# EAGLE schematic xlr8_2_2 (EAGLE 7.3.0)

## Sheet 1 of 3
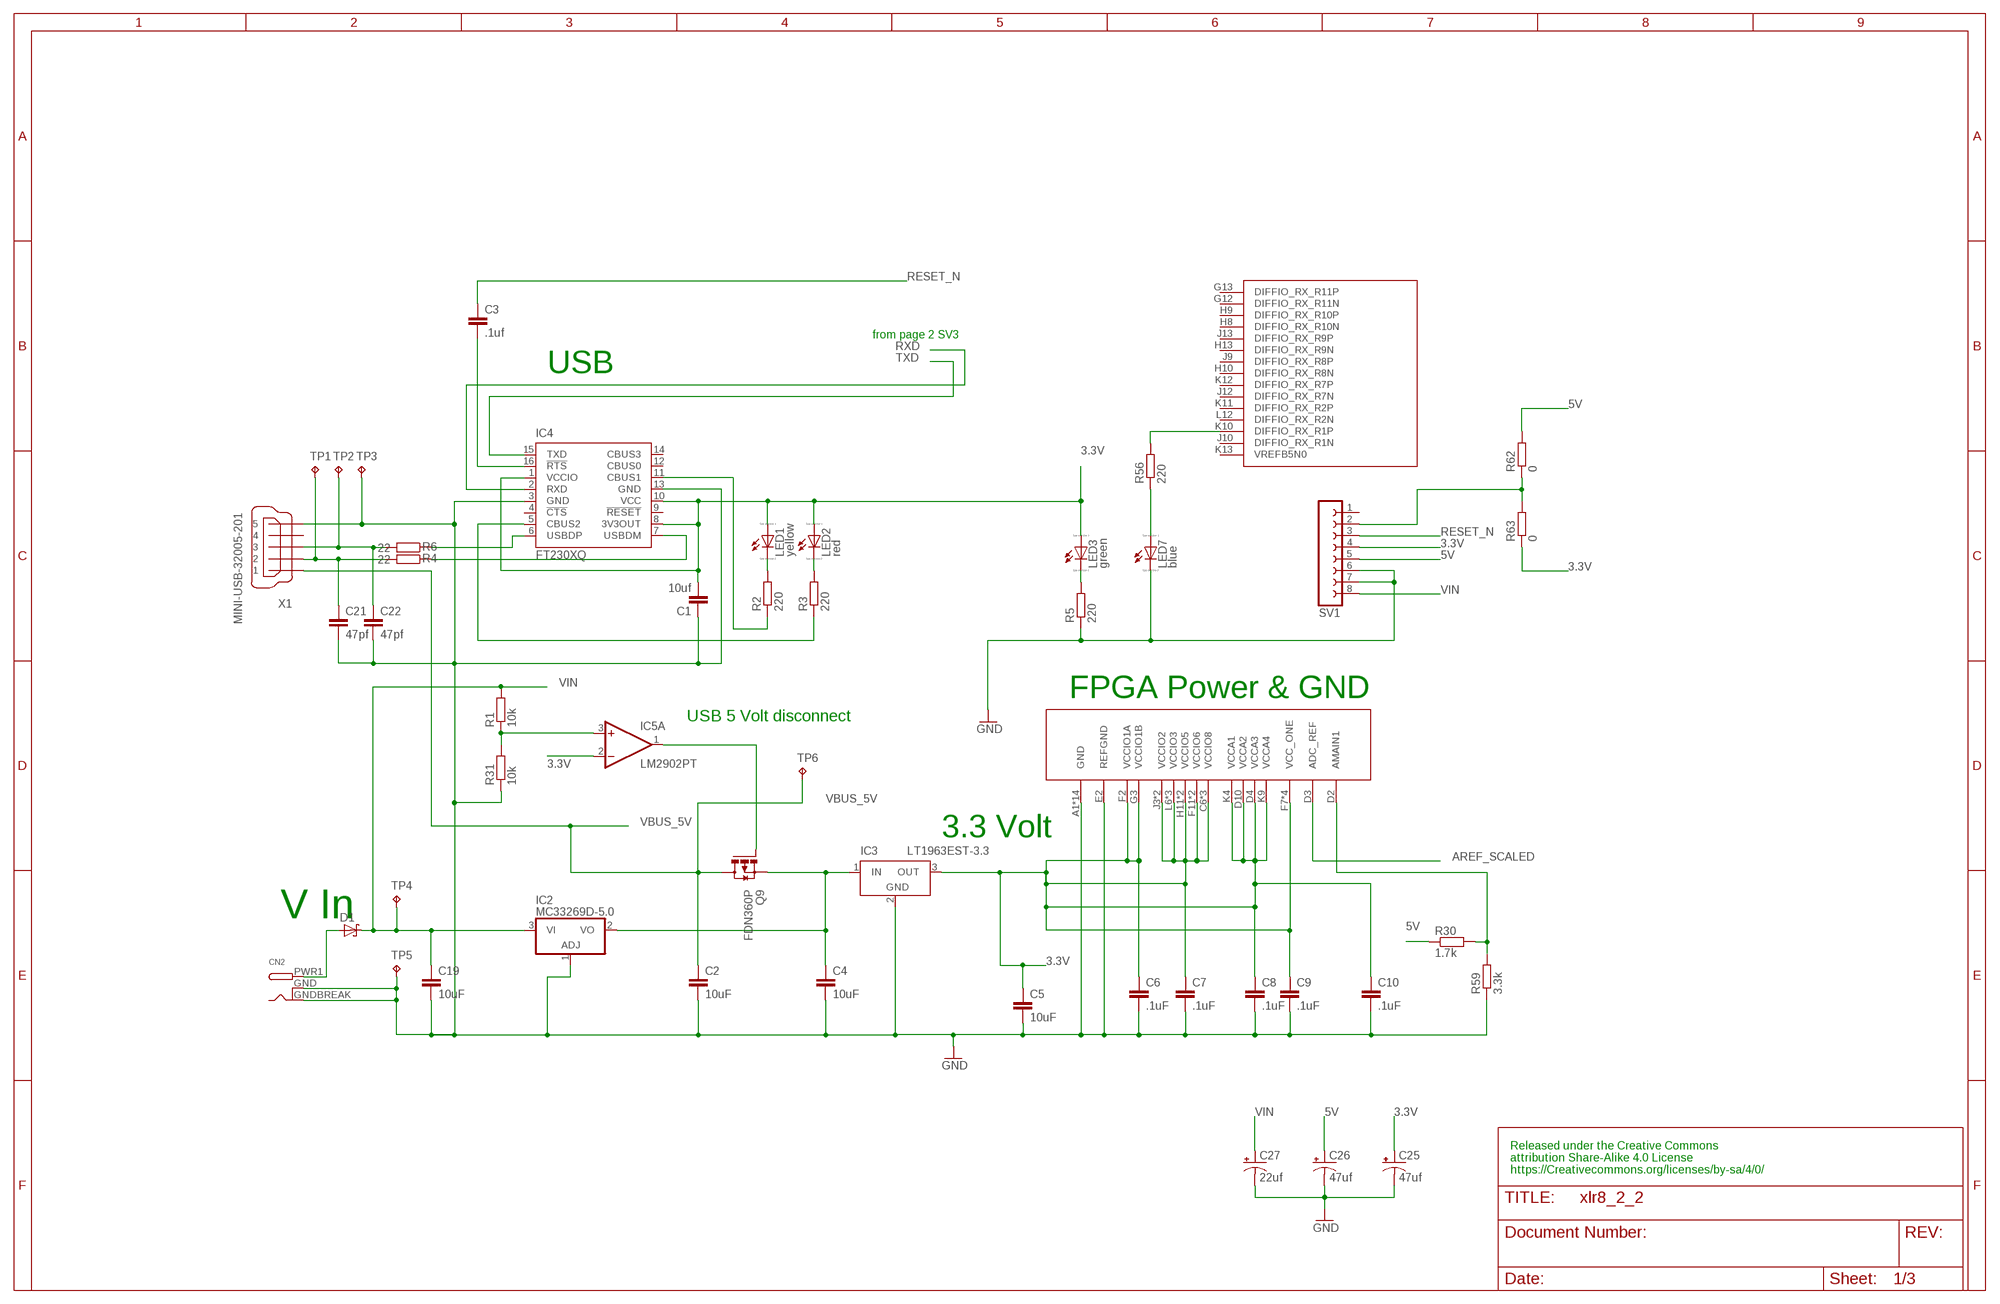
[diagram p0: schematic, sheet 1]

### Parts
C1  10uf  C-EUC0402  [C0402]
C2  10uF  C-EUC0402  [C0402]
C3  .1uf  C-EUC0402  [C0402]
C4  10uF  C-EUC0402  [C0402]
C5  10uF  C-EUC0402  [C0402]
C6  .1uF  C-EUC0402  [C0402]
C7  .1uF  C-EUC0402  [C0402]
C8  .1uF  C-EUC0402  [C0402]
C9  .1uF  C-EUC0402  [C0402]
C10  .1uF  C-EUC0402  [C0402]
C19  10uF  C-EUC0402  [C0402]
C21  47pf  C-EUC0402  [C0402]
C22  47pf  C-EUC0402  [C0402]
C25  47uf  CPOL-USB  [PANASONIC_B]
C26  47uf  CPOL-USB  [PANASONIC_B]
C27  22uf  CPOL-USB  [PANASONIC_B]
CN2  DCBARRELSMT  [DCJACK_2MM_SMT]
D1  SCHOTTKY-DIODESMD  [SMB]
IC2  MC33269D-5.0  [DPACK]
IC3  LT1963EST-3.3  [SOT223]
IC4  FT230XQ  [QFN16]
IC5  LM2902PT  [SSOP14]
LED1  yellow  LED_ESML0603  [LED_SML0603]
LED2  red  LED_ESML0603  [LED_SML0603]
LED3  green  LED_ESML0603  [LED_SML0603]
LED7  blue  LED_ESML0603  [LED_SML0603]
Q9  FDN360P  [SUPER-SOT3]
R1  10k  R-EU_R0402  [R0402]
R2  220  R-EU_R0402  [R0402]
R3  220  R-EU_R0402  [R0402]
R4  22  R-EU_R0402  [R0402]
R5  220  R-EU_R0402  [R0402]
R6  22  R-EU_R0402  [R0402]
R30  1.7k  R-EU_R0402  [R0402]
R31  10k  R-EU_R0402  [R0402]
R56  220  R-EU_R0402  [R0402]
R59  3.3k  R-EU_R0402  [R0402]
R62  0  R-EU_R0402  [R0402]
R63  0  R-EU_R0402  [R0402]
SV1  FE08-1  [FE08]
TP1  TPB2,54  [B2,54]
TP2  TPB2,54  [B2,54]
TP3  TPB2,54  [B2,54]
TP4  TPB2,54  [B2,54]
TP5  TPB2,54  [B2,54]
TP6  TPB2,54  [B2,54]
U1  10M08SA  [UBGA_169]
X1  MINI-USB-32005-201  [32005-201]

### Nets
3.3V: C1.2 C5.1 C6.1 C7.1 C8.1 C9.1 C10.1 C25.+ IC3.3(OUT) IC4.1(VCCIO) IC4.8(3V3OUT) IC4.10(VCC) IC5.2(A:-IN) LED1.A LED2.A LED3.A R63.1 SV1.4 U1.C6(VCCIO8) U1.C7(VCCIO8) U1.C8(VCCIO8) U1.D4(VCCA3) U1.D10(VCCA2) U1.F2(VCCIO1A) U1.F7(VCC_ONE) U1.F11(VCCIO6) U1.G3(VCCIO1B) U1.G6(VCC_ONE) U1.G8(VCC_ONE) U1.G11(VCCIO6) U1.H7(VCC_ONE) U1.H11(VCCIO5) U1.J3(VCCIO2) U1.J11(VCCIO5) U1.K3(VCCIO2) U1.K4(VCCA1) U1.K9(VCCA4) U1.L6(VCCIO3) U1.L7(VCCIO3) U1.L8(VCCIO3) ; also sheet 2,3
5V: C4.1 C26.+ IC2.2(VO) IC3.1(IN) Q9.2(S) R30.1 R62.2 SV1.5 ; also sheet 2
AREF_SCALED: U1.D3(ADC_REF) ; also sheet 2
GND: C1.1 C2.2 C4.2 C5.2 C6.2 C7.2 C8.2 C9.2 C10.2 C19.2 C21.2 C22.2 C25.- C26.- C27.- CN2.GND(GNDBREAK) CN2.GNDBREAK(GND) IC2.1(ADJ) IC3.2(GND) IC4.3(GND) IC4.13(GND) LED7.C R5.1 R31.1 R59.1 SV1.6 SV1.7 TP3.TP TP5.TP U1.A1(GND) U1.A13(GND) U1.B8(GND) U1.C3(GND) U1.D5(GND) U1.E2(REFGND) U1.E11(GND) U1.F3(GND) U1.G7(GND) U1.H12(GND) U1.J4(GND) U1.L9(GND) U1.M6(GND) U1.N1(GND) U1.N13(GND) X1.5 ; also sheet 2,3
N$6: C21.1 R4.2 TP1.TP X1.2
N$7: C22.1 R6.2 TP2.TP X1.3
N$16: LED1.C R2.2
N$20: IC4.7(USBDM) R4.1
N$21: IC4.6(USBDP) R6.1
N$23: IC4.11(CBUS1) R2.1
N$24: IC4.5(CBUS2) R3.1
N$29: CN2.PWR1(PWR) D1.A
N$36: LED7.A R56.1
N$47: IC5.1(A:OUT) Q9.1(G)
N$58: R30.2 R59.2 U1.D2(AMAIN1)
N$62: LED2.C R3.2
N$63: LED3.C R5.2
N$69: C3.2 IC4.16(!RTS)
N$72: IC5.3(A:+IN) R1.1 R31.2
N$80: R56.2 U1.K10(DIFFIO_RX_R1P)
N$81: R62.1 R63.2 SV1.2
RESET_N: C3.1 SV1.3 ; also sheet 2,3
RXD: IC4.2(RXD) ; also sheet 2
TXD: IC4.15(TXD) ; also sheet 2
VBUS_5V: C2.1 Q9.3(D) TP6.TP X1.1
VIN: C19.1 C27.+ D1.C IC2.3(VI) R1.2 SV1.8 TP4.TP
Unconnected: IC4.4(!CTS) IC4.9(!RESET) IC4.12(CBUS0) IC4.14(CBUS3) SV1.1 U1.G12(DIFFIO_RX_R11N) U1.G13(DIFFIO_RX_R11P) U1.H8(DIFFIO_RX_R10N) U1.H9(DIFFIO_RX_R10P) U1.H10(DIFFIO_RX_R8N) U1.H13(DIFFIO_RX_R9N) U1.J9(DIFFIO_RX_R8P) U1.J10(DIFFIO_RX_R1N) U1.J12(DIFFIO_RX_R7N) U1.J13(DIFFIO_RX_R9P) U1.K11(DIFFIO_RX_R2P) U1.K12(DIFFIO_RX_R7P) U1.K13(VREFB5N0) U1.L12(DIFFIO_RX_R2N) X1.4

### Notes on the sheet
- from page 2 SV3
- USB
- FPGA Power & GND
- USB 5 Volt disconnect
- 3.3 Volt
- V In
- Released under the Creative Commons
  attribution Share-Alike 4.0 License
  https://Creativecommons.org/licenses/by-sa/4/0/

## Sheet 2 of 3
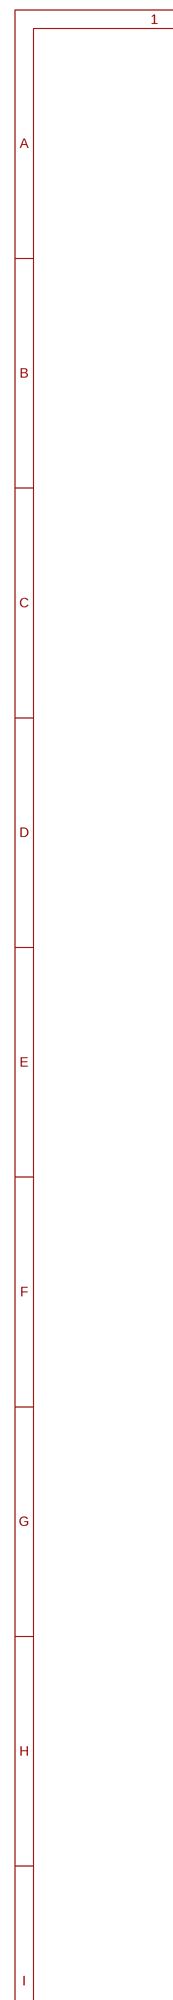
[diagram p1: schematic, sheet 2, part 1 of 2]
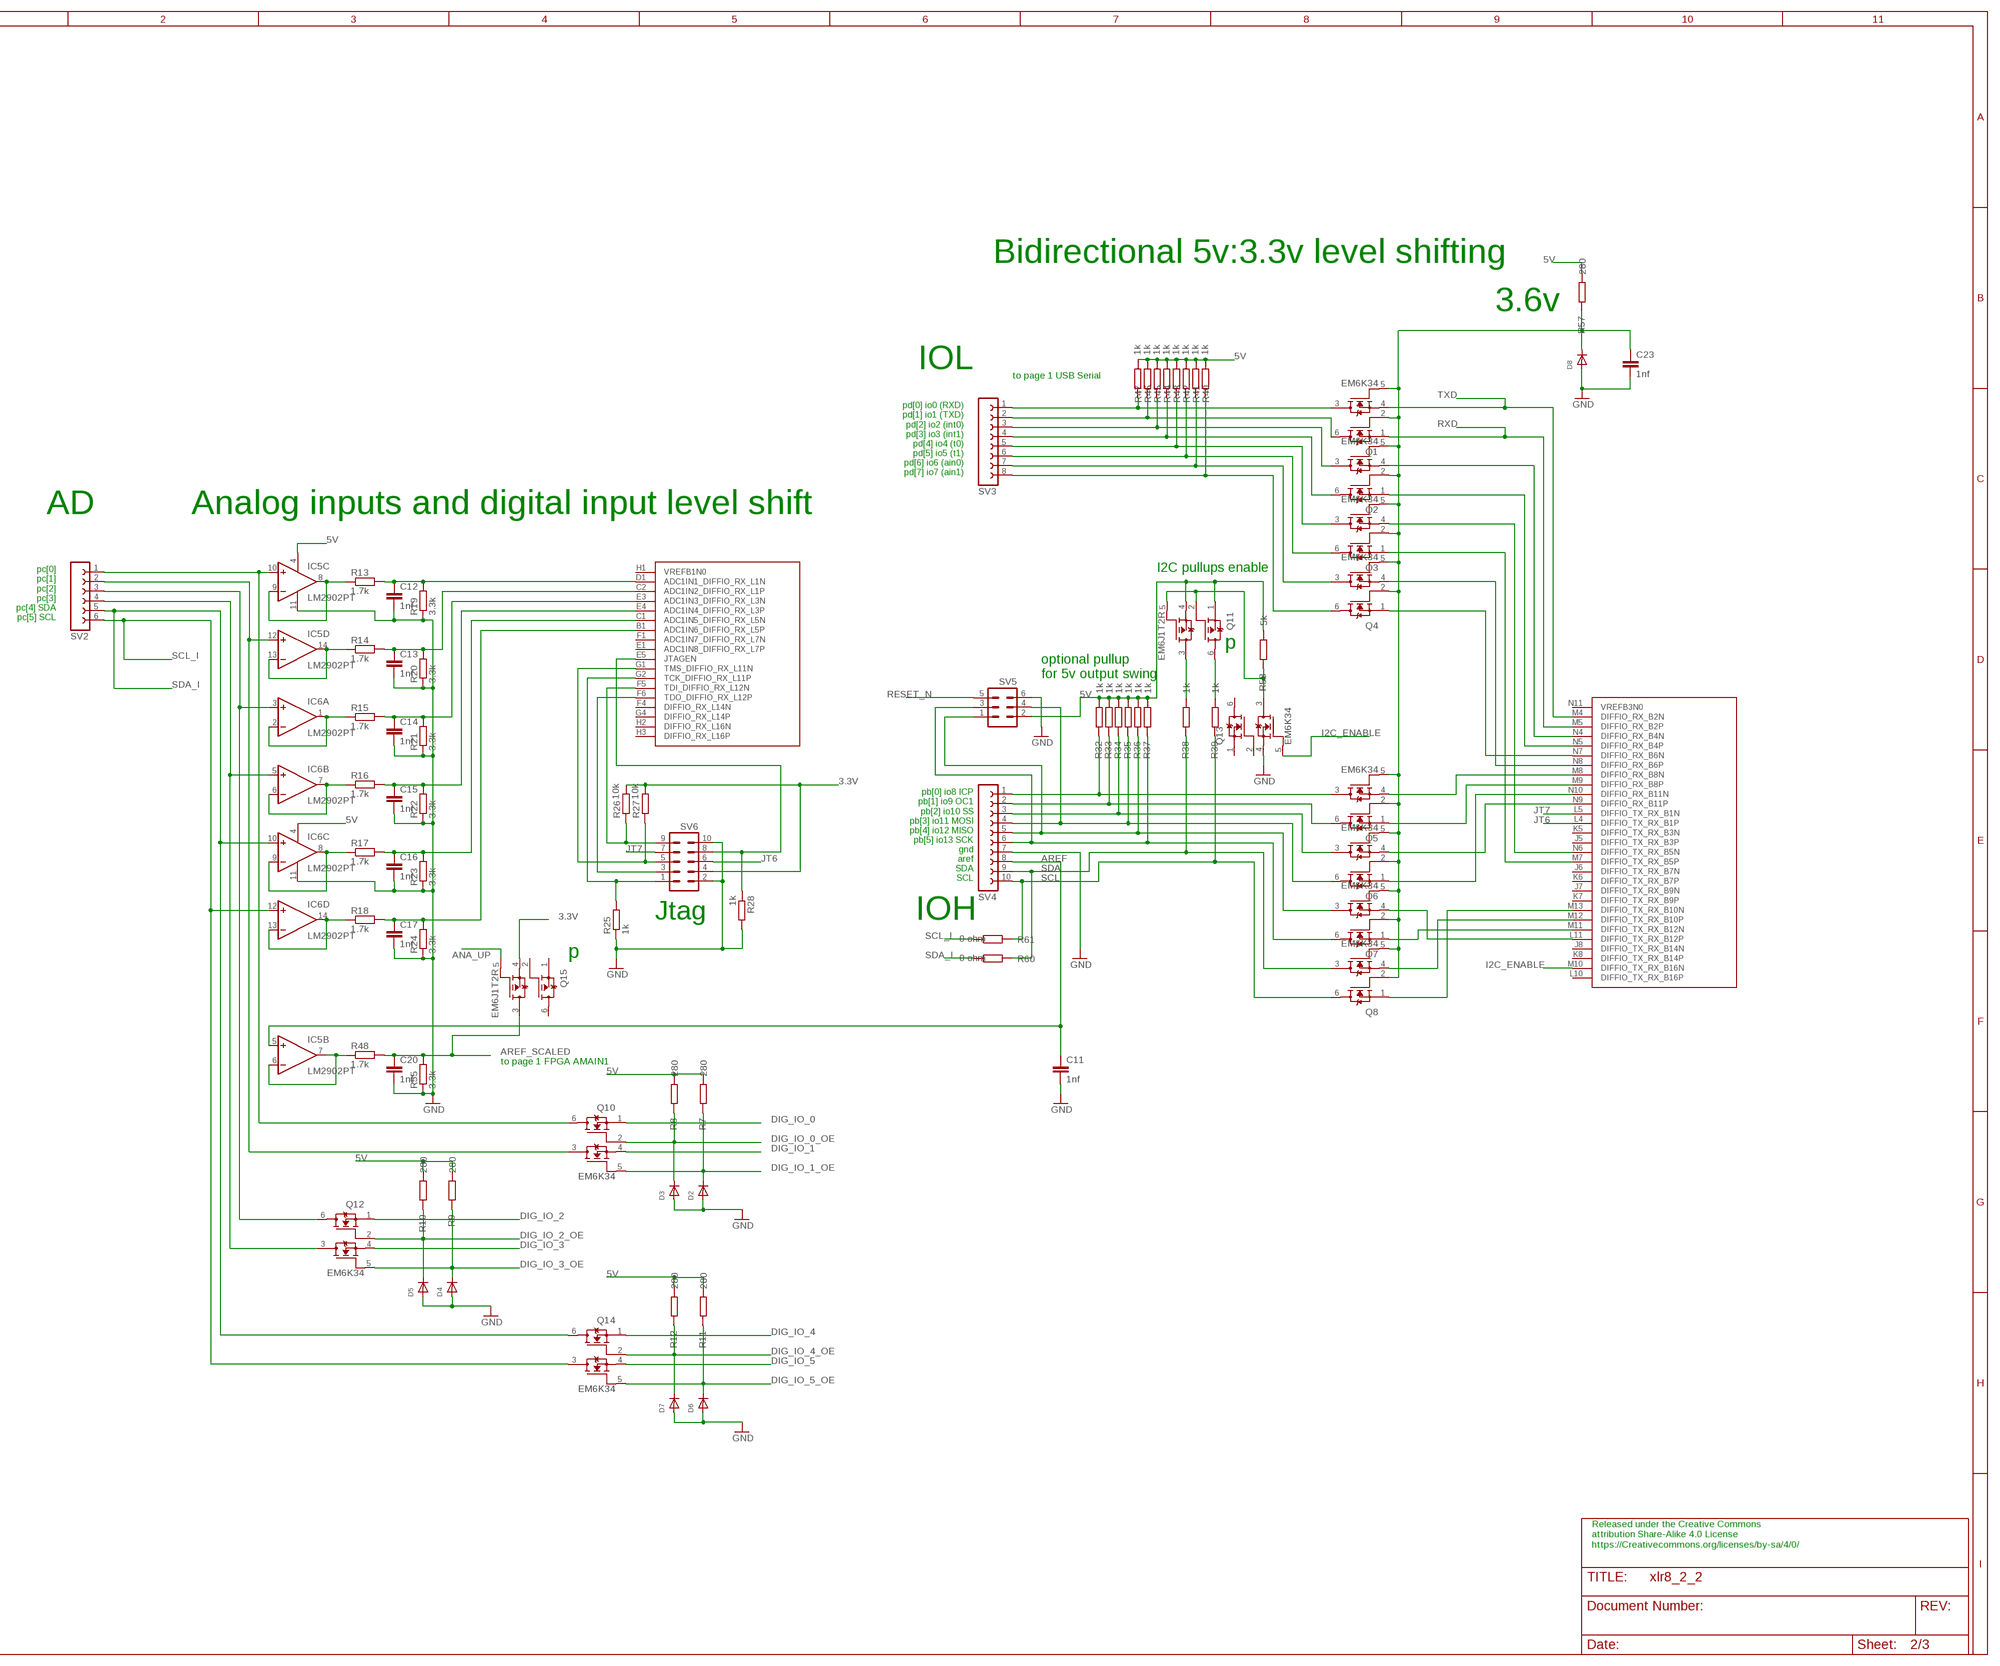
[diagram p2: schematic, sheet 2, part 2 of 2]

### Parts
C11  1nf  C-EUC0402  [C0402]
C12  1nf  C-EUC0402  [C0402]
C13  1nf  C-EUC0402  [C0402]
C14  1nf  C-EUC0402  [C0402]
C15  1nf  C-EUC0402  [C0402]
C16  1nf  C-EUC0402  [C0402]
C17  1nf  C-EUC0402  [C0402]
C20  1nf  C-EUC0402  [C0402]
C23  1nf  C-EUC0402  [C0402]
D2  DIODESOD-323F  [SOD-323F]
D3  DIODESOD-323F  [SOD-323F]
D4  DIODESOD-323F  [SOD-323F]
D5  DIODESOD-323F  [SOD-323F]
D6  DIODESOD-323F  [SOD-323F]
D7  DIODESOD-323F  [SOD-323F]
D8  DIODESOD-323F  [SOD-323F]
IC6  LM2902PT  [SSOP14]
Q1  EM6K34  EM6K34T2CR  [SOT-563]
Q2  EM6K34  EM6K34T2CR  [SOT-563]
Q3  EM6K34  EM6K34T2CR  [SOT-563]
Q4  EM6K34  EM6K34T2CR  [SOT-563]
Q5  EM6K34  EM6K34T2CR  [SOT-563]
Q6  EM6K34  EM6K34T2CR  [SOT-563]
Q7  EM6K34  EM6K34T2CR  [SOT-563]
Q8  EM6K34  EM6K34T2CR  [SOT-563]
Q10  EM6K34  EM6K34T2CR  [SOT-563]
Q11  EM6J1T2R  [SOT-563]
Q12  EM6K34  EM6K34T2CR  [SOT-563]
Q13  EM6K34  EM6K34T2CR  [SOT-563]
Q14  EM6K34  EM6K34T2CR  [SOT-563]
Q15  EM6J1T2R  [SOT-563]
R7  280  R-EU_R0402  [R0402]
R8  280  R-EU_R0402  [R0402]
R9  280  R-EU_R0402  [R0402]
R10  280  R-EU_R0402  [R0402]
R11  280  R-EU_R0402  [R0402]
R12  280  R-EU_R0402  [R0402]
R13  1.7k  R-EU_R0402  [R0402]
R14  1.7k  R-EU_R0402  [R0402]
R15  1.7k  R-EU_R0402  [R0402]
R16  1.7k  R-EU_R0402  [R0402]
R17  1.7k  R-EU_R0402  [R0402]
R18  1.7k  R-EU_R0402  [R0402]
R19  3.3k  R-EU_R0402  [R0402]
R20  3.3k  R-EU_R0402  [R0402]
R21  3.3k  R-EU_R0402  [R0402]
R22  3.3k  R-EU_R0402  [R0402]
R23  3.3k  R-EU_R0402  [R0402]
R24  3.3k  R-EU_R0402  [R0402]
R25  1k  R-EU_R0402  [R0402]
R26  10k  R-EU_R0402  [R0402]
R27  10k  R-EU_R0402  [R0402]
R28  1k  R-EU_R0402  [R0402]
R32  1k  R-EU_R0402  [R0402]
R33  1k  R-EU_R0402  [R0402]
R34  1k  R-EU_R0402  [R0402]
R35  1k  R-EU_R0402  [R0402]
R36  1k  R-EU_R0402  [R0402]
R37  1k  R-EU_R0402  [R0402]
R38  1k  R-EU_R0402  [R0402]
R39  1k  R-EU_R0402  [R0402]
R40  1k  R-EU_R0402  [R0402]
R41  1k  R-EU_R0402  [R0402]
R42  1k  R-EU_R0402  [R0402]
R43  1k  R-EU_R0402  [R0402]
R44  1k  R-EU_R0402  [R0402]
R45  1k  R-EU_R0402  [R0402]
R46  1k  R-EU_R0402  [R0402]
R47  1k  R-EU_R0402  [R0402]
R48  1.7k  R-EU_R0402  [R0402]
R55  3.3k  R-EU_R0402  [R0402]
R57  280  R-EU_R0402  [R0402]
R58  5k  R-EU_R0402  [R0402]
R60  0 ohm  R-EU_R0402  [R0402]
R61  0 ohm  R-EU_R0402  [R0402]
SV2  FE06-1  [FE06]
SV3  FE08-1  [FE08]
SV4  FE10-1  [FE10]
SV5  MA03-2  [MA03-2]
SV6  MA05-2  [MA05-2]

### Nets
3.3V: Q15.4(S2) R26.2 R27.2 SV6.4 ; also sheet 1,3
5V: IC5.4(P:V+) IC6.4(P:V+) Q11.1(S1) Q11.4(S2) R7.1 R8.1 R9.1 R10.1 R11.1 R12.1 R32.1 R33.1 R34.1 R35.1 R36.1 R37.1 R40.2 R41.2 R42.2 R43.2 R44.2 R45.2 R46.2 R47.2 R57.1 R58.1 SV5.2 ; also sheet 1
ANA_CMP_REF: Q4.3(D2) R41.1 SV3.7
ANA_UP: Q15.5(G2) ; also sheet 3
AREF: C11.1 IC5.5(B:+IN) SV4.8
AREF_SCALED: C20.1 Q15.3(D2) R48.2 R55.2 ; also sheet 1
DIG_IO_0: Q10.1(S1) ; also sheet 3
DIG_IO_0_OE: D3.C Q10.2(G1) R8.2 ; also sheet 3
DIG_IO_1: Q10.4(S2) ; also sheet 3
DIG_IO_1_OE: D2.C Q10.5(G2) R7.2 ; also sheet 3
DIG_IO_2: Q12.1(S1) ; also sheet 3
DIG_IO_2_OE: D5.C Q12.2(G1) R10.2 ; also sheet 3
DIG_IO_3: Q12.4(S2) ; also sheet 3
DIG_IO_3_OE: D4.C Q12.5(G2) R9.2 ; also sheet 3
DIG_IO_4: Q14.1(S1) ; also sheet 3
DIG_IO_4_OE: D7.C Q14.2(G1) R12.2 ; also sheet 3
DIG_IO_5: Q14.4(S2) ; also sheet 3
DIG_IO_5_OE: D6.C Q14.5(G2) R11.2 ; also sheet 3
GND: C11.2 C12.2 C13.2 C14.2 C15.2 C16.2 C17.2 C20.2 C23.2 D2.A D3.A D4.A D5.A D6.A D7.A D8.A IC5.11(P:V-) IC6.11(P:V-) Q13.4(S2) R19.1 R20.1 R21.1 R22.1 R23.1 R24.1 R25.1 R28.2 R55.1 SV4.7 SV5.6 SV6.2 SV6.10 ; also sheet 1,3
I2C_ENABLE: Q13.5(G2) U1.M10(DIFFIO_TX_RX_B16N)
JT6: SV6.6 U1.L4(DIFFIO_TX_RX_B1P)
JT7: SV6.7 U1.L5(DIFFIO_TX_RX_B1N)
N$1: R28.1 SV6.8 U1.E5(JTAGEN)
N$2: R27.1 SV6.5 U1.G1(TMS_DIFFIO_RX_L11N)
N$3: R25.2 SV6.1 U1.G2(TCK_DIFFIO_RX_L11P)
N$4: R26.1 SV6.9 U1.F5(TDI_DIFFIO_RX_L12N)
N$5: SV6.3 U1.F6(TDO_DIFFIO_RX_L12P)
N$8: IC5.8(C:OUT) IC5.9(C:-IN) R13.1
N$9: IC5.13(D:-IN) IC5.14(D:OUT) R14.1
N$10: IC6.1(A:OUT) IC6.2(A:-IN) R15.1
N$11: IC6.6(B:-IN) IC6.7(B:OUT) R16.1
N$12: IC6.8(C:OUT) IC6.9(C:-IN) R17.1
N$13: IC6.13(D:-IN) IC6.14(D:OUT) R18.1
N$14: C12.1 R13.2 R19.2 U1.D1(ADC1IN1_DIFFIO_RX_L1N)
N$15: C13.1 R14.2 R20.2 U1.C2(ADC1IN2_DIFFIO_RX_L1P)
N$17: C14.1 R15.2 R21.2 U1.E3(ADC1IN3_DIFFIO_RX_L3N)
N$19: C16.1 R17.2 R23.2 U1.C1(ADC1IN5_DIFFIO_RX_L5N)
N$22: C17.1 R18.2 R24.2 U1.B1(ADC1IN6_DIFFIO_RX_L5P)
N$25: Q5.3(D2) R32.2 SV4.1
N$26: Q5.6(D1) R33.2 SV4.2
N$27: IC5.10(C:+IN) Q10.6(D1) SV2.1
N$28: Q7.1(S1) U1.M11(DIFFIO_TX_RX_B12N)
N$30: Q4.1(S1) U1.N7(DIFFIO_RX_B6N)
N$31: Q6.6(D1) R35.2 SV4.4 SV5.4
N$32: Q6.1(S1) U1.N10(DIFFIO_RX_B11N)
N$33: IC5.6(B:-IN) IC5.7(B:OUT) R48.1
N$34: Q4.4(S2) U1.N8(DIFFIO_RX_B6P)
N$35: Q3.1(S1) U1.M7(DIFFIO_TX_RX_B5P)
N$38: Q3.4(S2) U1.N6(DIFFIO_TX_RX_B5N)
N$39: Q7.3(D2) R36.2 SV4.5 SV5.1
N$40: Q6.4(S2) U1.N9(DIFFIO_RX_B11P)
N$41: Q7.6(D1) R37.2 SV4.6 SV5.3
N$42: Q5.1(S1) U1.M9(DIFFIO_RX_B8P)
N$43: Q2.3(D2) R45.1 SV3.3
N$44: Q2.1(S1) U1.N5(DIFFIO_RX_B4P)
N$45: Q2.4(S2) U1.N4(DIFFIO_RX_B4N)
N$46: Q2.6(D1) R44.1 SV3.4
N$48: Q6.3(D2) R34.2 SV4.3
N$49: Q3.3(D2) R43.1 SV3.5
N$51: Q3.6(D1) R42.1 SV3.6
N$53: Q11.3(D2) R38.1
N$54: Q11.6(D1) R39.1
N$55: Q1.3(D2) R47.1 SV3.1
N$56: IC6.5(B:+IN) Q12.3(D2) SV2.4
N$57: IC6.3(A:+IN) Q12.6(D1) SV2.3
N$61: Q5.4(S2) U1.M8(DIFFIO_RX_B8N)
N$64: Q1.6(D1) R46.1 SV3.2
N$65: Q4.6(D1) R40.1 SV3.8
N$66: Q8.4(S2) U1.M12(DIFFIO_TX_RX_B10P)
N$68: Q8.1(S1) U1.M13(DIFFIO_TX_RX_B10N)
N$70: C15.1 R16.2 R22.2 U1.E4(ADC1IN4_DIFFIO_RX_L3P)
N$73: C23.1 D8.C Q1.2(G1) Q1.5(G2) Q2.2(G1) Q2.5(G2) Q3.2(G1) Q3.5(G2) Q4.2(G1) Q4.5(G2) Q5.2(G1) Q5.5(G2) Q6.2(G1) Q6.5(G2) Q7.2(G1) Q7.5(G2) Q8.2(G1) Q8.5(G2) R57.2
N$75: IC5.12(D:+IN) Q10.3(D2) SV2.2
N$82: Q11.2(G1) Q11.5(G2) Q13.3(D2) R58.2
N$103: Q7.4(S2) U1.L11(DIFFIO_TX_RX_B12P)
RESET_N: SV5.5 ; also sheet 1,3
RXD: Q1.1(S1) U1.M5(DIFFIO_RX_B2P) ; also sheet 1
SCL: Q8.6(D1) R39.2 R61.2 SV4.10
SCL_I: IC6.12(D:+IN) Q14.3(D2) R61.1 SV2.6
SDA: Q8.3(D2) R38.2 R60.2 SV4.9
SDA_I: IC6.10(C:+IN) Q14.6(D1) R60.1 SV2.5
TXD: Q1.4(S2) U1.M4(DIFFIO_RX_B2N) ; also sheet 1
Unconnected: Q13.1(S1) Q13.2(G1) Q13.6(D1) Q15.1(S1) Q15.2(G1) Q15.6(D1) U1.E1(ADC1IN8_DIFFIO_RX_L7P) U1.F1(ADC1IN7_DIFFIO_RX_L7N) U1.F4(DIFFIO_RX_L14N) U1.G4(DIFFIO_RX_L14P) U1.H1(VREFB1N0) U1.H2(DIFFIO_RX_L16N) U1.H3(DIFFIO_RX_L16P) U1.J5(DIFFIO_TX_RX_B3P) U1.J6(DIFFIO_TX_RX_B7N) U1.J7(DIFFIO_TX_RX_B9N) U1.J8(DIFFIO_TX_RX_B14N) U1.K5(DIFFIO_TX_RX_B3N) U1.K6(DIFFIO_TX_RX_B7P) U1.K7(DIFFIO_TX_RX_B9P) U1.K8(DIFFIO_TX_RX_B14P) U1.L10(DIFFIO_TX_RX_B16P) U1.N11(VREFB3N0)

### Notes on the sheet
- Bidirectional 5v:3.3v level shifting
- 3.6v
- IOL
- to page 1 USB Serial
- pd[0] io0 (RXD)
  pd[1] io1 (TXD)
  pd[2] io2 (int0)
  pd[3] io3 (int1)
  pd[4] io4 (t0)
  pd[5] io5 (t1)
  pd[6] io6 (ain0)
  pd[7] io7 (ain1)
- AD | Analog inputs and digital input level shift
- I2C pullups enable
- pc[0]
  pc[1]
  pc[2]
  pc[3]
  pc[4] SDA
  pc[5] SCL
- p
- optional pullup
  for 5v output swing
- pb[0] io8 ICP
  pb[1] io9 OC1
  pb[2] io10 SS
  pb[3] io11 MOSI
  pb[4] io12 MISO
  pb[5] io13 SCK
  gnd
  aref
  SDA
  SCL
- Jtag | IOH
- p
- to page 1 FPGA AMAIN1
- Released under the Creative Commons
  attribution Share-Alike 4.0 License
  https://Creativecommons.org/licenses/by-sa/4/0/

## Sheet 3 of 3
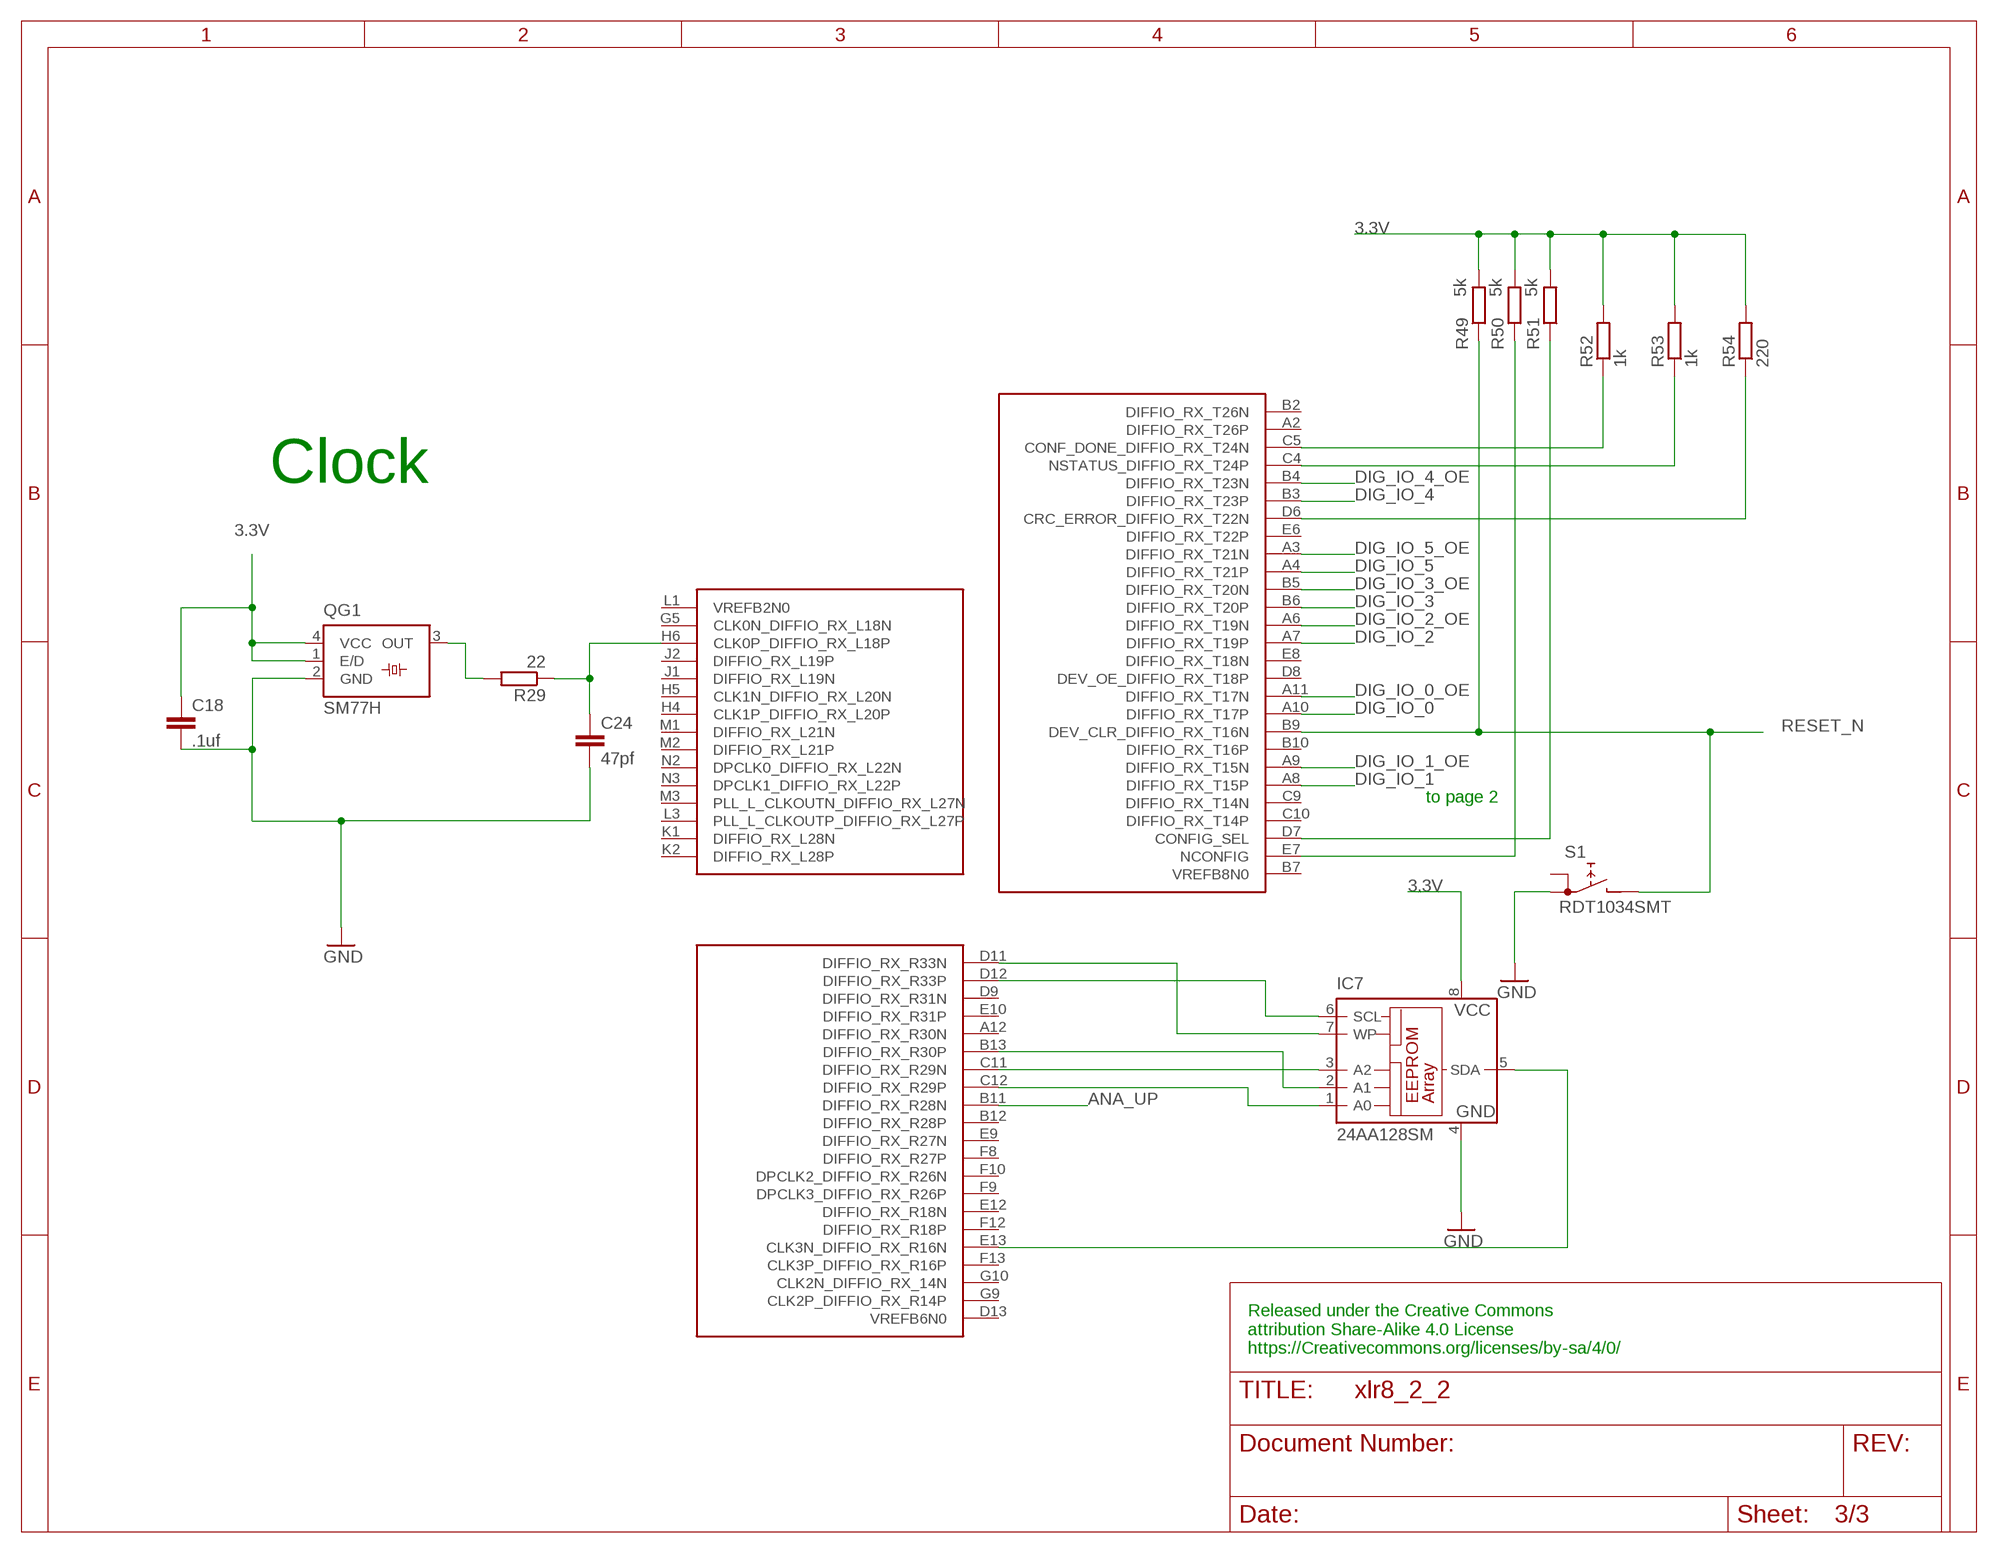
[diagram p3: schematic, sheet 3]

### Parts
C18  .1uf  C-EUC0402  [C0402]
C24  47pf  C-EUC0402  [C0402]
IC7  24AA128SM  [SO-08M]
QG1  SM77H  [SM77H]
R29  22  R-EU_R0402  [R0402]
R49  5k  R-EU_R0402  [R0402]
R50  5k  R-EU_R0402  [R0402]
R51  5k  R-EU_R0402  [R0402]
R52  1k  R-EU_R0402  [R0402]
R53  1k  R-EU_R0402  [R0402]
R54  220  R-EU_R0402  [R0402]
S1  RDT1034SMT  [6MM_SMT]

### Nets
3.3V: C18.1 IC7.8(VCC) QG1.1(E/D) QG1.4(VCC) R49.2 R50.2 R51.2 R52.2 R53.2 R54.2 ; also sheet 1,2
ANA_UP: U1.B11(DIFFIO_RX_R28N) ; also sheet 2
DIG_IO_0: U1.A10(DIFFIO_RX_T17P) ; also sheet 2
DIG_IO_0_OE: U1.A11(DIFFIO_RX_T17N) ; also sheet 2
DIG_IO_1: U1.A8(DIFFIO_RX_T15P) ; also sheet 2
DIG_IO_1_OE: U1.A9(DIFFIO_RX_T15N) ; also sheet 2
DIG_IO_2: U1.A7(DIFFIO_RX_T19P) ; also sheet 2
DIG_IO_2_OE: U1.A6(DIFFIO_RX_T19N) ; also sheet 2
DIG_IO_3: U1.B6(DIFFIO_RX_T20P) ; also sheet 2
DIG_IO_3_OE: U1.B5(DIFFIO_RX_T20N) ; also sheet 2
DIG_IO_4: U1.B3(DIFFIO_RX_T23P) ; also sheet 2
DIG_IO_4_OE: U1.B4(DIFFIO_RX_T23N) ; also sheet 2
DIG_IO_5: U1.A4(DIFFIO_RX_T21P) ; also sheet 2
DIG_IO_5_OE: U1.A3(DIFFIO_RX_T21N) ; also sheet 2
GND: C18.2 C24.2 IC7.4(GND) QG1.2(GND) S1.2(A1) ; also sheet 1,2
N$18: R52.1 U1.C5(CONF_DONE_DIFFIO_RX_T24N)
N$37: QG1.3(OUT) R29.2
N$50: IC7.1(A0) U1.C12(DIFFIO_RX_R29P)
N$52: IC7.2(A1) U1.B13(DIFFIO_RX_R30P)
N$59: R53.1 U1.C4(NSTATUS_DIFFIO_RX_T24P)
N$60: C24.1 R29.1 U1.H6(CLK0P_DIFFIO_RX_L18P)
N$67: R51.1 U1.D7(CONFIG_SEL)
N$71: R54.1 U1.D6(CRC_ERROR_DIFFIO_RX_T22N)
N$74: IC7.3(A2) U1.C11(DIFFIO_RX_R29N)
N$77: IC7.5(SDA) U1.E13(CLK3N_DIFFIO_RX_R16N)
N$78: IC7.6(SCL) U1.D12(DIFFIO_RX_R33P)
N$79: IC7.7(WP) U1.D11(DIFFIO_RX_R33N)
NCONFIG: R50.1 U1.E7(NCONFIG)
RESET_N: R49.1 S1.4(B) U1.B9(DEV_CLR_DIFFIO_RX_T16N) ; also sheet 1,2
Unconnected: S1.1(A) U1.A2(DIFFIO_RX_T26P) U1.A12(DIFFIO_RX_R30N) U1.B2(DIFFIO_RX_T26N) U1.B7(VREFB8N0) U1.B10(DIFFIO_RX_T16P) U1.B12(DIFFIO_RX_R28P) U1.C9(DIFFIO_RX_T14N) U1.C10(DIFFIO_RX_T14P) U1.D8(DEV_OE_DIFFIO_RX_T18P) U1.D9(DIFFIO_RX_R31N) U1.D13(VREFB6N0) U1.E6(DIFFIO_RX_T22P) U1.E8(DIFFIO_RX_T18N) U1.E9(DIFFIO_RX_R27N) U1.E10(DIFFIO_RX_R31P) U1.E12(DIFFIO_RX_R18N) U1.F8(DIFFIO_RX_R27P) U1.F9(DPCLK3_DIFFIO_RX_R26P) U1.F10(DPCLK2_DIFFIO_RX_R26N) U1.F12(DIFFIO_RX_R18P) U1.F13(CLK3P_DIFFIO_RX_R16P) U1.G5(CLK0N_DIFFIO_RX_L18N) U1.G9(CLK2P_DIFFIO_RX_R14P) U1.G10(CLK2N_DIFFIO_RX_14N) U1.H4(CLK1P_DIFFIO_RX_L20P) U1.H5(CLK1N_DIFFIO_RX_L20N) U1.J1(DIFFIO_RX_L19N) U1.J2(DIFFIO_RX_L19P) U1.K1(DIFFIO_RX_L28N) U1.K2(DIFFIO_RX_L28P) U1.L1(VREFB2N0) U1.L3(PLL_L_CLKOUTP_DIFFIO_RX_L27P) U1.M1(DIFFIO_RX_L21N) U1.M2(DIFFIO_RX_L21P) U1.M3(PLL_L_CLKOUTN_DIFFIO_RX_L27N) U1.N2(DPCLK0_DIFFIO_RX_L22N) U1.N3(DPCLK1_DIFFIO_RX_L22P)

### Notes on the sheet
- Clock
- to page 2
- Released under the Creative Commons
  attribution Share-Alike 4.0 License
  https://Creativecommons.org/licenses/by-sa/4/0/

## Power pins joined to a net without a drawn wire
GND: IC3.4(GND)

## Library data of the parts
C1-C24 = rcl:C-EU: CAPACITOR, European symbol
C25-C27 = adafruit:CPOL-US: POLARIZED CAPACITOR, American symbol
CN2 = adafruit:DCBARREL: 2.0mm DC Barrel Jack DCJACK_2MM_PTH - Through Hole Jack (4UConnector: 05537)
D1 = diode:SCHOTTKY-DIODE: Schottky Diode
D2-D8 = adafruit:DIODE: Diode
IC2 = linear:MC33269?*: Adjustable Output Low Dropout Voltage Regulator 800 mA Source: http://www.onsemi.com/pub/Collateral/MC33269-D.PDF
IC3 = linear-technology:LT1963EST: 1.5A, Low Noise, Fast Transient Response LDO Regulator Source: http://www.linear.com/pc/downloadDocument.do?navId=H0,C3,P2222,D3148; MPN: LT1963EST-3.3; OC_FARNELL: 1501032; OC_NEWARK: 57M7546
IC4 = ftdichip:FT230X: USB to BASIC UART IC Auto generated by make-symbol-device-package-bsdl.ulp Rev. 43 Source: Data sheet
IC5 IC6 = linear:LM2902: Low power quad operational amplifier Source: Data sgeet
IC7 = microchip:24*: Serial EEPROM I2C; MF: MICROCHIP; MPN: 24AA128-I/MS; OC_FARNELL: 1331285; OC_NEWARK: 92C6839
LED1-LED3 LED7 = eagle-ltspice:LED_E: LED; SPICEMODEL: NONE; SPICEPREFIX: D; SPICETYPE: diode
Q1-Q8 Q10 Q12-Q14 = Superion:EM6K34T2CR: OnSemi dual N-channel Small Signal MOSFET 20V 430mA Datasheet (from onsemi)
Q9 = transistor-power:FDN360P: Single P-Channel, PowerTrench (R) MOSFET Source: http://www.fairchildsemi.com/ds/FD/FDN360P.pdf
Q11 Q15 = Superion:EM6J1T2R: OnSemi dual P-channel Small Signal MOSFET 20V 430mA Datasheet (from onsemi)
QG1 = crystal:SM77H: 3.3V CMOS Clock Oscillator Source: www.pletronics.com .. sm77h%203.3v.pdf; OC_FARNELL: unknown; OC_NEWARK: unknown
R1-R63 = rcl:R-EU_: RESISTOR, European symbol
S1 = Superion:RDT1034: PUSH SWITCH www.radiohm.com
SV1 SV3 = con-lsta:FE08-1: FEMALE HEADER; OC_FARNELL: unknown; OC_NEWARK: unknown
SV2 = con-lsta:FE06-1: FEMALE HEADER; OC_FARNELL: unknown; OC_NEWARK: unknown
SV4 = con-lsta:FE10-1: FEMALE HEADER; OC_FARNELL: unknown; OC_NEWARK: unknown
SV5 = con-lstb:MA03-2: PIN HEADER; OC_FARNELL: unknown; OC_NEWARK: unknown
SV6 = con-lstb:MA05-2: PIN HEADER; OC_FARNELL: unknown; OC_NEWARK: unknown
TP1-TP6 = testpad:TP: Test pad
U1 = Superion:10M08SA
X1 = con-cypressindustries:MINI-USB-: MINI USB-B Conector Source: www.cypressindustries.com; OC_FARNELL: unknown; OC_NEWARK: unknown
